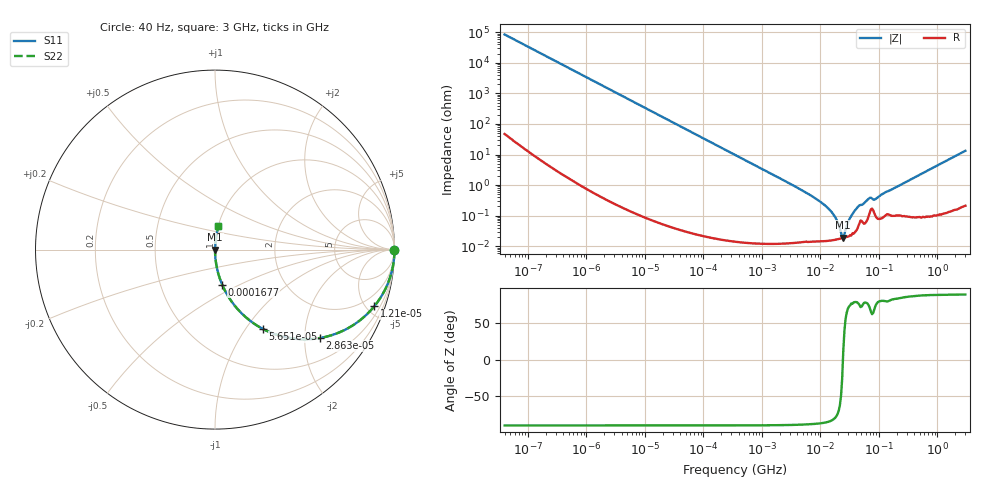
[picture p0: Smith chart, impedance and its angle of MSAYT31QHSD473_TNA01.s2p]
! MSAYT31QHSD473_TNA01  S-PARAMETER MODEL  ( General Type )
! Model Generated by TAIYO YUDEN Corporation (http://www.ty-top.com)
! Version 2.0
! TAIYO YUDEN Control No. 031016
! Copyright(c) 2003 TAIYO YUDEN CO.,LTD. All Rights Reserved.
! Product Description (link to TY-COMPAS)
! https://ds.yuden.co.jp/TYCOMPAS/or/detail?pn=MSAYT31QHSD473KTNA01&u=M
! Products Name : Multilayer Ceramic Capacitors
! Characteristics :
!  Capacitance : 0.047 uF , Rated Voltage : 25V
!  Case Size : 3.2 x 1.6 / 0.126 x 0.063 [mm/inch] , Thickness : 1.15 / 0.045 [mm/inch]
!  (Conditions: Temperature = 25 degC , DC Bias Current/Voltage = 0A / 0V)
! External Node Assignments :
!  1  o---| |---o  2
! GND o---------o GND
! Frequency Range : 40Hz  -  3GHz  [ 401 STEP ]
# MHz S RI R 50
! Freq[MHz].  S11 Real  S11 Imag  S21 Real  S21 Imag  S12 Real  S12 Imag  S22 Real  S22 Imag
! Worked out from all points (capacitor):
!   401 points, 40 Hz to 3 GHz, reference 50 ohm
!   read as one part in series: C = 46.8 nF near 44 Hz
!   lowest |Z| = 19.1 mohm at 24.56 MHz (marker M1)
!   series resonance near 24.23 MHz, so ESL is about 920 pH
!   S11 on the Smith chart (normalised r, x): 40 Hz: open; 12.1 kHz: 1.00, -5.62; 28.63 kHz: 1.00, -2.37; 56.51 kHz: 1.00, -1.20; 167.7 kHz: 1.00, -0.41; 3 GHz: 1.00, +0.27
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4e-05  1 -0.00118  2.04e-06 0.00118  2.04e-06 0.00118  1 -0.00118
0.000834  0.9994 -0.0245  0.000607 0.0245  0.000607 0.0245  0.9994 -0.0245
0.003895  0.987 -0.1131  0.013 0.1131  0.013 0.1131  0.987 -0.1131
0.012098  0.8875 -0.3159  0.1125 0.3159  0.1125 0.3159  0.8875 -0.3159
0.017386  0.7925 -0.4053  0.2075 0.4053  0.2075 0.4053  0.7925 -0.4053
0.028627  0.585 -0.4926  0.415 0.4926  0.415 0.4926  0.585 -0.4926
0.056505  0.2658 -0.4415  0.7342 0.4415  0.7342 0.4415  0.2658 -0.4415
0.093035  0.1179 -0.3222  0.8821 0.3222  0.8821 0.3222  0.1179 -0.3222
0.167721  0.0396 -0.1946  0.9604 0.1946  0.9604 0.1946  0.0396 -0.1946
0.362475  0.00885 -0.0929  0.9912 0.0929  0.9912 0.0929  0.00885 -0.0929
7.222098  0.000159 -0.00429  0.9998 0.00429  0.9998 0.00429  0.000159 -0.00429
11.36423  0.000151 -0.00234  0.9998 0.00234  0.9998 0.00234  0.000151 -0.00234
15.60822  0.000156 -0.00129  0.9998 0.00129  0.9998 0.00129  0.000156 -0.00129
18.71131  0.000165 -0.000734  0.9998 0.000734  0.9998 0.000734  0.000165 -0.000734
22.43131  0.000179 -0.000216  0.9998 0.000216  0.9998 0.000216  0.000179 -0.000216
24.56009  0.000187 4e-05  0.9998 -4e-05  0.9998 -4e-05  0.000187 4e-05
32.2371  0.000231 0.000826  0.9998 -0.000826  0.9998 -0.000826  0.000231 0.000826
44.27611  0.000451 0.00194  0.9995 -0.00194  0.9995 -0.00194  0.000451 0.00194
66.58224  0.000967 0.00344  0.999 -0.00344  0.999 -0.00344  0.000967 0.00344
87.39454  0.000976 0.00333  0.999 -0.00333  0.999 -0.00333  0.000976 0.00333
150.5692  0.00109 0.00646  0.9989 -0.00646  0.9989 -0.00646  0.00109 0.00646
3000  0.0193 0.1297  0.9807 -0.1297  0.9807 -0.1297  0.0193 0.1297
